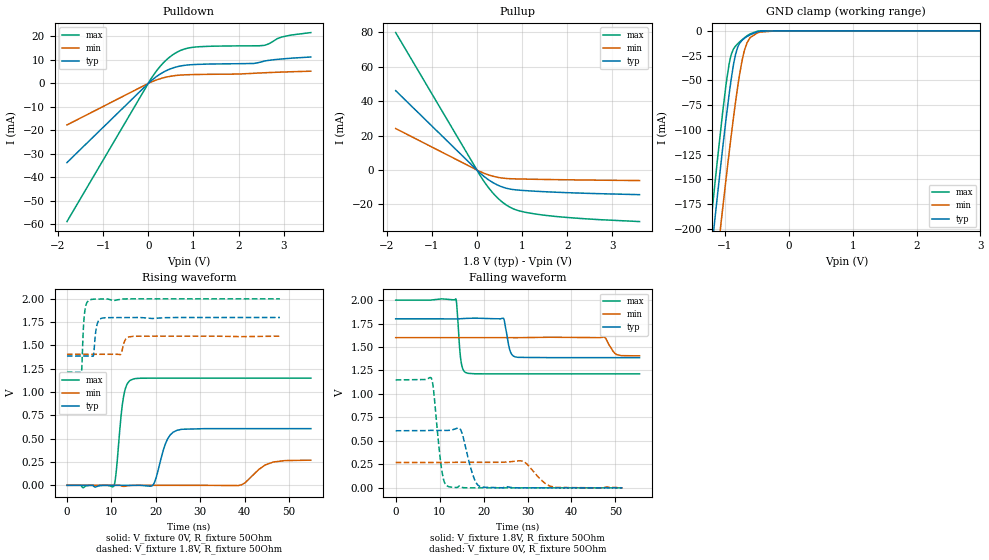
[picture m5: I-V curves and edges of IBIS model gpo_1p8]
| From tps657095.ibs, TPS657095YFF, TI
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|   gpo_1p8 Model
[Model]   gpo_1p8
Model_type   3-state
Polarity   Non-Inverting
Vmeas = 0.9
Vref = 0
Cref = 2pF
Rref = 200
|   typ   min   max
|   (nom PVT)   (fast PVT)   (slow PVT)
C_comp   6.950e-12   6.807e-12   7.251e-12
| Where nom  PVT is Nominal Process, 1.8V, 27C
|   Fast PVT is Strong Process,  2V, -40C
|   Slow PVT is Weak Process,   1.6V, 125C
[Voltage Range]   1.8   1.6   2
|Junction Temperature
[Temperature Range]   27   125   -40
[Pullup Reference]   1.8   1.6   2
[Pulldown Reference]   0   0   0
[Power Clamp Reference]   1.8   1.6   2
[GND Clamp Reference]   0   0   0
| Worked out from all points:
|   slope of the pulldown table from 0 to 0.27 V, typ, clamps not added: 66.6 ohm
|   slope of the pullup table from 0 to 0.27 V, typ, clamps not added: 45.6 ohm
|   GND clamp passes 1 mA (typ) near -0.49 V on its own axis
|   falling waveform, V_fixture 1.8V, R_fixture 50Ohm: 20-80 % time 1.01ns typ, 1.51ns min, 747ps max; typ from 1.8 V to 1.39 V
|   rising waveform, V_fixture 0V, R_fixture 50Ohm: 20-80 % time 2.24ns typ, 3.87ns min, 1.38ns max; typ from 0 V to 0.608 V
|   rising waveform, V_fixture 1.8V, R_fixture 50Ohm: 20-80 % time 609ps typ, 735ps min, 522ps max; typ from 1.39 V to 1.8 V
|   falling waveform, V_fixture 0V, R_fixture 50Ohm: 20-80 % time 2.05ns typ, 3.25ns min, 1.48ns max; typ from 0.608 V to 0 V
[Pulldown]
|   Voltage   I(typ)   I(min)   I(max)
-1.8V     -33.74mA   -17.71mA   -58.9mA
38.4mV    708.5uA    357.4uA    1.285mA
258mV     3.918mA    1.96mA     7.145mA
473.6mV   6.067mA    2.98mA     11.22mA
688mV     7.329mA    3.512mA    13.82mA
902.4mV   7.9mA      3.719mA    15.15mA
1.332V    8.241mA    3.872mA    15.81mA
2.338V    8.503mA    4.313mA    16.03mA
2.564V    9.481mA    4.53mA     16.21mA
2.672V    9.837mA    4.622mA    16.9mA
2.954V    10.42mA    4.832mA    19.77mA
3.6V      11.26mA    5.202mA    21.67mA
[GND Clamp]
|   Voltage   I(typ)   I(min)   I(max)
-1.8V     -601mA     -648mA     -578.6mA
-1.421V   -354.7mA   -410mA     -324.1mA
-1.2V     -216.2mA   -275.7mA   -181.2mA
-1.168V   -196.7mA   -256.6mA   -161.1mA
-1.124V   -170.1mA   -230.6mA   -134mA
-1.034V   -117.5mA   -178.5mA   -81.16mA
-914.4mV  -54.39mA   -112.4mA   -27.2mA
-833.4mV  -23.62mA   -71.47mA   -15.34mA
-732.8mV  -9.566mA   -30.31mA   -9.012mA
-606mV    -3.945mA   -6.819mA   -3.08mA
-180mV    -220.3nA   -6.289uA   -14.47nA
3.6V      0A         66.39nA    0A
[Pullup]
|   Voltage   I(typ)   I(min)   I(max)
-1.8V     46.15mA    24.12mA    79.91mA
84.8mV    -2.127mA   -1.081mA   -3.781mA
248mV     -5.526mA   -2.759mA   -9.983mA
352mV     -7.28mA    -3.582mA   -13.33mA
579.6mV   -10.02mA   -4.727mA   -19.02mA
688mV     -10.82mA   -4.977mA   -20.97mA
848mV     -11.48mA   -5.141mA   -22.99mA
1.332V    -12.38mA   -5.402mA   -25.71mA
2.308V    -13.43mA   -5.772mA   -28.19mA
3.6V      -14.31mA   -6.117mA   -29.95mA
[POWER Clamp]
|   Voltage   I(typ)   I(min)   I(max)
-1.8V     0A         0A         0A
0V        0A         0A         0A
3.6V      0A         0A         0A
[Ramp]
R_load = 50
|   typ   min   max
dV/dt_r   0.364885/2.22717e-09   0.162021/3.80762e-09   0.689856/1.37308e-09
dV/dt_f   0.247821/9.98403e-10   0.116619/1.50131e-09   0.471762/7.47129e-10
[Falling Waveform]
V_fixture = 1.8V
V_fixture_min = 1.6V
V_fixture_max = 2V
R_fixture = 50Ohm
|   Time   V(typ)   V(min)   V(max)
0s        1.8V       1.6V       2V
13.69ns   1.8V       1.6V       2.013V
14.9ns    1.802V     1.6V       1.338V
16.45ns   1.806V     1.6V       1.22V
24.48ns   1.808V     1.6V       1.214V
25.88ns   1.483V     1.6V       1.214V
27.16ns   1.396V     1.6V       1.214V
47.44ns   1.387V     1.605V     1.214V
50.06ns   1.387V     1.426V     1.214V
55.48ns   1.387V     1.406V     1.214V
[Rising Waveform]
V_fixture = 0V
V_fixture_min = 0V
V_fixture_max = 0V
R_fixture = 50Ohm
|   Time   V(typ)   V(min)   V(max)
0s        140.1pV    8.162nV    76.29pV
10.55ns   -15.23uV   -5.135uV   -8.992mV
12.77ns   -203.5uV   -11.16mV   959.2mV
14.97ns   -163.3uV   -365.9uV   1.141V
19.51ns   13.6mV     -4.028uV   1.15V
22.18ns   447.4mV    -3.798uV   1.15V
24.75ns   589.9mV    -9.383uV   1.15V
38.55ns   608.1mV    -2.728mV   1.15V
46.48ns   608.1mV    250.2mV    1.15V
54.9ns    608.1mV    269.9mV    1.15V
[Rising Waveform]
V_fixture = 1.8V
V_fixture_min = 1.6V
V_fixture_max = 2V
R_fixture = 50Ohm
|   Time   V(typ)   V(min)   V(max)
0s        1.387V     1.406V     1.214V
3.244ns   1.387V     1.406V     1.212V
4.012ns   1.387V     1.406V     1.866V
5.447ns   1.387V     1.406V     1.994V
5.969ns   1.394V     1.406V     1.996V
6.814ns   1.732V     1.406V     1.998V
7.768ns   1.792V     1.406V     1.998V
12.05ns   1.799V     1.403V     1.996V
14.97ns   1.8V       1.599V     2V
47.94ns   1.8V       1.6V       2V
[Falling Waveform]
V_fixture = 0V
V_fixture_min = 0V
V_fixture_max = 0V
R_fixture = 50Ohm
|   Time   V(typ)   V(min)   V(max)
0s        608.1mV    270mV      1.15V
8.123ns   612mV      270mV      1.169V
10.55ns   611.7mV    270mV      169.7mV
11.99ns   612mV      270.6mV    14.13mV
14.74ns   621.6mV    272.2mV    10.21mV
17.43ns   154.3mV    271.9mV    211.9uV
19.11ns   15.78mV    271.8mV    125.9uV
28.85ns   160.8uV    284.6mV    16.62uV
36.59ns   41.39uV    4.87mV     4.79uV
51.61ns   5.426uV    172.9uV    1.168uV
